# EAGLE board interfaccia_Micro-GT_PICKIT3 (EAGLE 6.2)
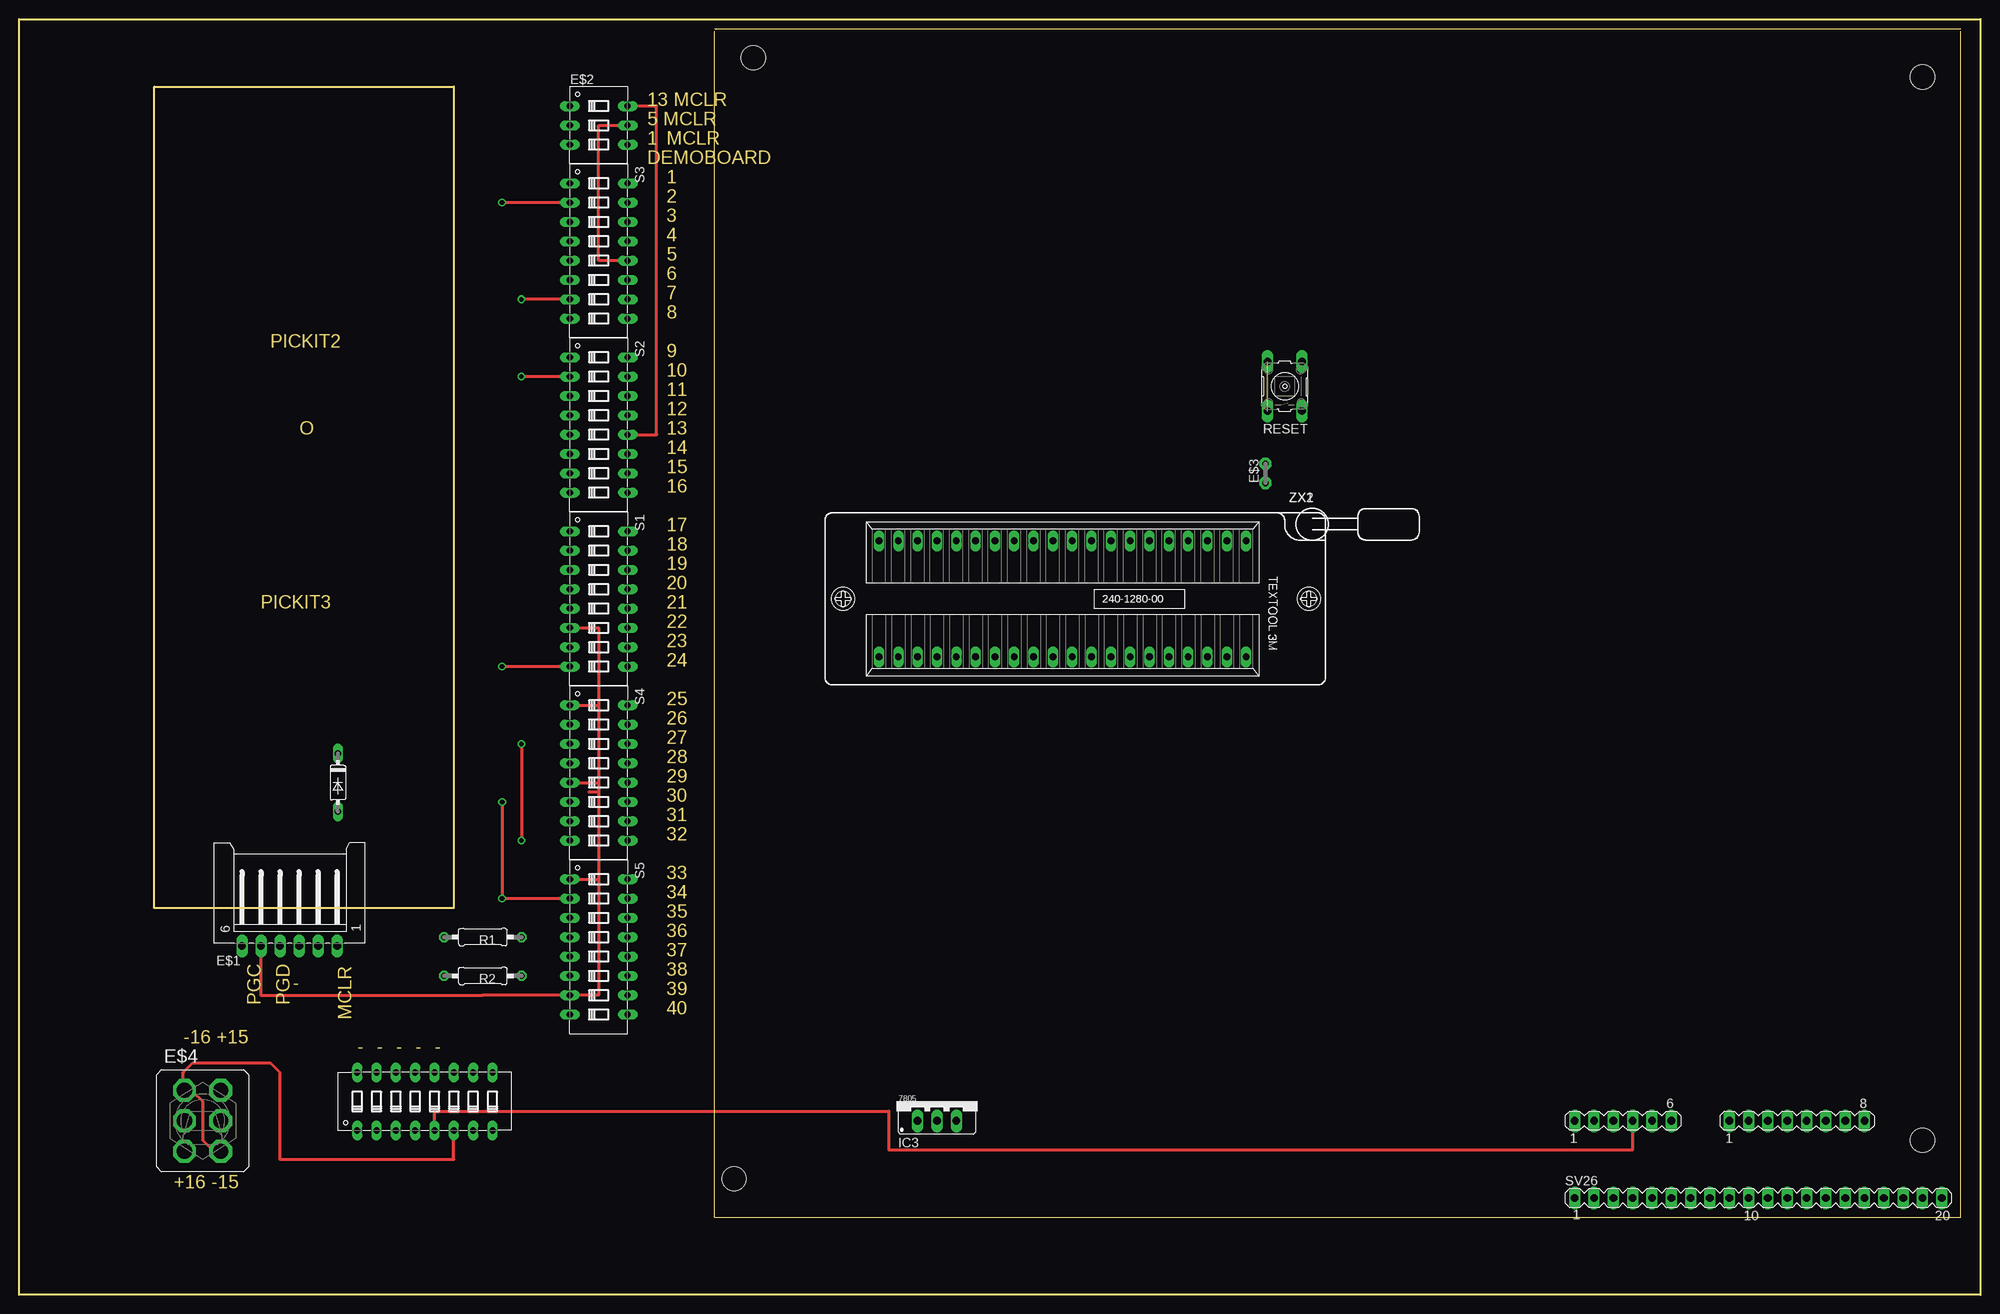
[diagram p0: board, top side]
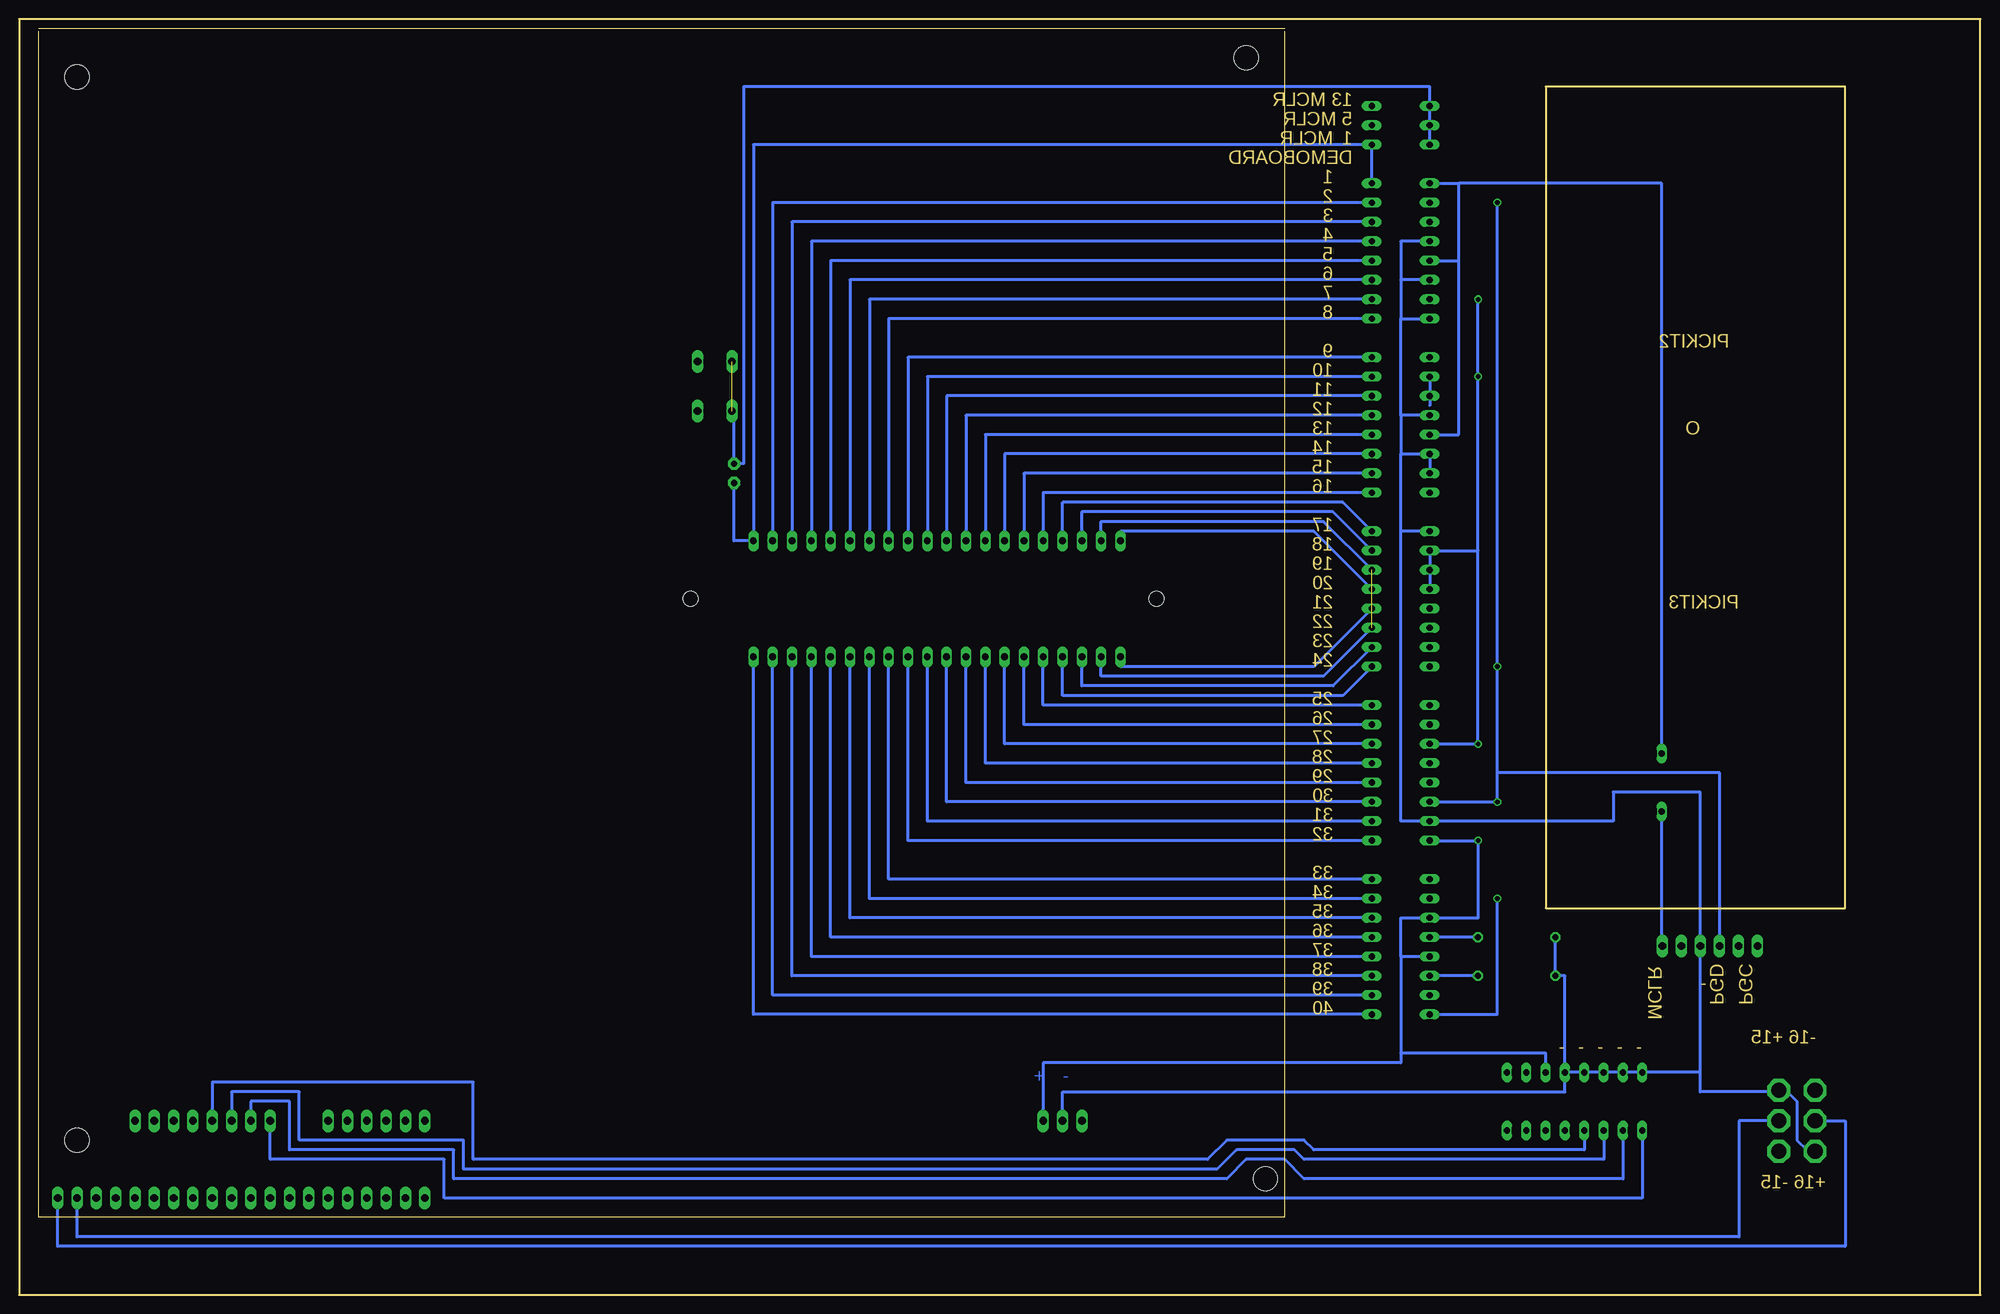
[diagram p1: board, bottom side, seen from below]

Size 257.81 x 167.64 mm. Coordinates in mm from the lower left corner, seen from the top.
Outline: 91.44,10.16 255.25,10.16 255.25,166.04
Outline: 91.42,10.16 91.42,166.04
Outline: 91.44,166.37 255.25,166.37
Outline: 0,0 0,167.64 257.81,167.64 257.81,0 0,0
Outline: 17.78,50.8 17.78,158.75 57.15,158.75 57.15,50.8 17.78,50.8
Copper layers (1*16): Top 0.035mm / dielectric 1.5mm / Bottom 0.035mm
Design rules: minimum track width 10mil, minimum drill 24mil, track to track 8mil, track to pad 8mil, pad to pad 8mil, via to via 8mil, smd to smd 8mil, copper to edge 40mil, drill to drill 8mil, minimum pad ring 10mil, minimum via ring 8mil, stop-mask expansion 4mil, vias tented up to drill 0mil, thermal gap 10mil
Holes 3.2 mm at 250.19,160.02 250.19,20.32 93.98,15.24 96.52,162.56

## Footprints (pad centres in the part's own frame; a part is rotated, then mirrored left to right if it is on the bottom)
DO35-7 = drill 0.813 long: A 3.81,0; C -3.81,0
L06P = drill 1.016 long: 1 6.25,-6.25; 2 3.75,-6.25; 3 1.25,-6.25; 4 -1.25,-6.25; 5 -3.75,-6.25; 6 -6.25,-6.25
DIP03YL = drill 0.813 long: 1 -2.54,-3.81; 2 0,-3.81; 3 2.54,-3.81; 4 2.54,3.81; 5 0,3.81; 6 -2.54,3.81
03 = drill 0.813 pad 1.6 octagon: 1 0,0; 2 2.54,0
320-938 = drill 2.007 octagon: 1 -2.388,4.013; 2 -2.388,0; 3 -2.388,-4.013; 4 2.388,4.013; 5 2.388,0; 6 2.388,-4.013
78XXS = drill 1.016 long: GND 0,-2.54; IN -2.54,-2.54; OUT 2.54,-2.54
0207/10 = drill 0.813 octagon: 1 -5.08,0; 2 5.08,0
B3F-10XX = drill 1.016 long: 1 -3.251,2.261; 2 3.251,2.261; 3 -3.251,-2.261; 4 3.251,-2.261
DIP08YL = drill 0.813 long: 1 -8.89,-3.81; 2 -6.35,-3.81; 3 -3.81,-3.81; 4 -1.27,-3.81; 5 1.27,-3.81; 6 3.81,-3.81; 7 6.35,-3.81; 8 8.89,-3.81; 9 8.89,3.81; 10 6.35,3.81; 11 3.81,3.81; 12 1.27,3.81; 13 -1.27,3.81; 14 -3.81,3.81; 15 -6.35,3.81; 16 -8.89,3.81
MA20-1 = drill 1.016 long: 1 -24.13,0; 2 -21.59,0; 3 -19.05,0; 4 -16.51,0; 5 -13.97,0; 6 -11.43,0; 7 -8.89,0; 8 -6.35,0; 9 -3.81,0; 10 -1.27,0; 11 1.27,0; 12 3.81,0; 13 6.35,0; 14 8.89,0; 15 11.43,0; 16 13.97,0; 17 16.51,0; 18 19.05,0; 19 21.59,0; 20 24.13,0
MA06-1 = drill 1.016 long: 1 -6.35,0; 2 -3.81,0; 3 -1.27,0; 4 1.27,0; 5 3.81,0; 6 6.35,0
MA08-1 = drill 1.016 long: 1 -8.89,0; 2 -6.35,0; 3 -3.81,0; 4 -1.27,0; 5 1.27,0; 6 3.81,0; 7 6.35,0; 8 8.89,0
240-1280-00-0602J = drill 0.9 long: 1 -24.13,-7.62; 2 -21.59,-7.62; 3 -19.05,-7.62; 4 -16.51,-7.62; 5 -13.97,-7.62; 6 -11.43,-7.62; 7 -8.89,-7.62; 8 -6.35,-7.62; 9 -3.81,-7.62; 10 -1.27,-7.62; 11 1.27,-7.62; 12 3.81,-7.62; 13 6.35,-7.62; 14 8.89,-7.62; 15 11.43,-7.62; 16 13.97,-7.62; 17 16.51,-7.62; 18 19.05,-7.62; 19 21.59,-7.62; 20 24.13,-7.62; 21 24.13,7.62; 22 21.59,7.62; 23 19.05,7.62; 24 16.51,7.62; 25 13.97,7.62; 26 11.43,7.62; 27 8.89,7.62; 28 6.35,7.62; 29 3.81,7.62; 30 1.27,7.62; 31 -1.27,7.62; 32 -3.81,7.62; 33 -6.35,7.62; 34 -8.89,7.62; 35 -11.43,7.62; 36 -13.97,7.62; 37 -16.51,7.62; 38 -19.05,7.62; 39 -21.59,7.62; 40 -24.13,7.62 | hole 2: 28.86,0; -32.36,0

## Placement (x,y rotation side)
D1  1N4007  [DO35-7]  41.91,67.31 270 top
E$1  [L06P]  35.56,52.07 0 top
E$2  [DIP03YL]  76.2,153.67 270 top
E$3  [03]  163.83,106.68 90 top
E$4  [320-938]  24.13,22.86 0 top
IC3  [78XXS]  120.65,25.4 0 top
R1  1K  [0207/10]  60.96,46.99 0 top
R2  1K  [0207/10]  60.96,41.91 0 top
RESET  [B3F-10XX]  166.37,119.38 90 top
S1  [DIP08YL]  76.2,91.44 270 top
S2  [DIP08YL]  76.2,114.3 270 top
S3  [DIP08YL]  76.2,137.16 270 top
S4  [DIP08YL]  76.2,68.58 270 top
S5  [DIP08YL]  76.2,45.72 270 top
S6  [DIP08YL]  53.34,25.4 0 top
SV26  [MA20-1]  228.6,12.7 0 top
SV27  [MA06-1]  210.82,22.86 0 top
SV28  [MA08-1]  233.68,22.86 0 top
ZX1  240-1280-00-0602J  [240-1280-00-0602J]  137.16,91.44 180 top
ZX2  240-1280-00-0602J  [240-1280-00-0602J]  137.16,91.44 180 top

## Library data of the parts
D1 = diode
E$1 = con-amp-mt
E$2 S1-S6 = switch-dil
E$3 = jumper
E$4 = switch
IC3 = v-reg
R1 R2 = resistor
RESET = switch-omron
SV26-SV28 = con-lstb
ZX1 ZX2 = con-3m

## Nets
N$87: RESET.1 RESET.2
N$124: ZX2.18
N$125: ZX2.23
N$128: ZX2.26
S$1: S5.9 ZX1.40
S$2: S5.10
S$3: S5.11 ZX1.38
S$4: S5.12 ZX1.37
S$5: S5.13 ZX1.36
S$6: S5.14 ZX1.35
S$7: S5.15 ZX1.34
S$8: S5.16 ZX1.33
S$9: S4.9 ZX1.32
S$10: S4.10 ZX1.31
S$12: S4.11 ZX1.30
S$13: S4.12 ZX1.29
S$14: S4.13 ZX1.28
S$15: S4.14 ZX1.27
S$16: S4.15 ZX1.26
S$18: S4.16 ZX1.25
S$19: ZX1.17
S$20: S1.10 ZX1.23
S$21: S1.11 ZX1.19 ZX1.22
S$22: S1.12 ZX1.20 ZX1.21
S$23: ZX1.18
S$24: S2.9 ZX1.16
S$25: S2.10 ZX1.15
S$26: S2.11 ZX1.14
S$27: E$2.6 S2.12 ZX1.13
S$28: S2.13 ZX1.12
S$29: S2.14 ZX1.11
S$30: S2.15 ZX1.10
S$31: S2.16 ZX1.9
S$32: S3.9 ZX1.8
S$33: S3.10 ZX1.7
S$34: S3.11 ZX1.6
S$35: E$2.5 S3.12 ZX1.5
S$36: S3.13 ZX1.4
S$37: S3.14 ZX1.3
S$38: S3.15 ZX1.2
S$39: S6.5 SV27.4
S$40: S3.5
S$41: D1.C S2.5 S3.1
S$43: R1.2 S5.4
S$44: R2.2 S5.6
S$46: E$2.1 E$2.3 E$3.2
S$47: S1.9 ZX1.24
S$48: IC3.OUT S1.2 S1.4 S2.2 S3.7 S4.3 S4.8 S5.3 S5.5 S6.11
S$49: S1.8 S3.2 S4.6 S5.2 S5.8
S$50: S1.6 S4.1
S$51: IC3.GND R1.1 R2.1 S1.1 S2.4 S2.6 S2.7 S3.4 S3.6 S3.8 S4.7 S6.12 S6.16
S$52: S4.5 S5.1 S5.7
S$53: E$2.4 E$3.1 S3.16 ZX1.1
S$56: S6.6
S$57: S6.1 SV28.1
S$58: S6.2 SV28.2
S$59: S6.3 SV28.3
S$60: S6.4 SV28.4
S$61: SV26.19
S$62: SV26.20

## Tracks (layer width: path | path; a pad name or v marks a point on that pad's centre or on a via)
N$87  (1 unrouted)
S$1
  Bottom 0.406: S5.9 161.29,36.83 ZX1.40
S$2
  Bottom 0.406: S5.10 158.75,39.37 158.75,83.82
S$3
  Bottom 0.406: S5.11 156.21,41.91 ZX1.38
S$4
  Bottom 0.406: S5.12 153.67,44.45 ZX1.37
S$5
  Bottom 0.406: S5.13 151.13,46.99 ZX1.36
S$6
  Bottom 0.406: S5.14 148.59,49.53 ZX1.35
S$7
  Bottom 0.406: S5.15 146.05,52.07 ZX1.34
S$8
  Bottom 0.406: S5.16 143.51,54.61 ZX1.33
S$9
  Bottom 0.406: S4.9 140.97,59.69 ZX1.32
S$10
  Bottom 0.406: S4.10 138.43,62.23 ZX1.31
S$12
  Bottom 0.406: S4.11 135.89,64.77 ZX1.30
S$13
  Bottom 0.406: S4.12 133.35,67.31 ZX1.29
S$14
  Bottom 0.406: S4.13 130.81,69.85 ZX1.28
S$15
  Bottom 0.406: S4.14 128.27,72.39 ZX1.27
S$16
  Bottom 0.406: S4.15 125.73,74.93 ZX1.26
S$18
  Bottom 0.406: S4.16 123.19,77.47 ZX1.25
S$19
  Bottom 0.406: 80.01,100.33 83.82,104.14 120.65,104.14 ZX1.17
S$20
  Bottom 0.406: S1.10 85.09,80.01 118.11,80.01 ZX1.23
S$21  (1 unrouted)
  Bottom 0.406: S1.11 86.36,81.28 115.57,81.28 ZX1.22 | 80.01,95.25 86.36,101.6 115.57,101.6 ZX1.19
S$22  (1 unrouted)
  Bottom 0.406: S1.12 87.63,82.55 113.03,82.55 ZX1.21 | 80.01,92.71 87.63,100.33 113.03,100.33 ZX1.20
S$23
  Bottom 0.406: 80.01,97.79 85.09,102.87 118.11,102.87 ZX1.18
S$24
  Bottom 0.406: S2.9 123.19,105.41 ZX1.16
S$25
  Bottom 0.406: S2.10 125.73,107.95 ZX1.15
S$26
  Bottom 0.406: S2.11 128.27,110.49 ZX1.14
S$27
  Top 0.406: S2.12 83.82,113.03 83.82,156.21 E$2.6
  Bottom 0.406: S2.12 130.81,113.03 ZX1.13
S$28
  Bottom 0.406: S2.13 133.35,115.57 ZX1.12
S$29
  Bottom 0.406: S2.14 135.89,118.11 ZX1.11
S$30
  Bottom 0.406: S2.15 138.43,120.65 ZX1.10
S$31
  Bottom 0.406: S2.16 140.97,123.19 ZX1.9
S$32
  Bottom 0.406: S3.9 143.51,128.27 ZX1.8
S$33
  Bottom 0.406: S3.10 146.05,130.81 ZX1.7
S$34
  Bottom 0.406: S3.11 148.59,133.35 ZX1.6
S$35
  Top 0.406: S3.12 76.2,135.89 76.2,153.67 E$2.5
  Bottom 0.406: S3.12 151.13,135.89 ZX1.5
S$36
  Bottom 0.406: S3.13 153.67,138.43 ZX1.4
S$37
  Bottom 0.406: S3.14 156.21,140.97 ZX1.3
S$38
  Bottom 0.406: S3.15 158.75,143.51 ZX1.2
S$39
  Top 0.406: S6.5 54.61,24.13 114.3,24.13 114.3,19.05 212.09,19.05 SV27.4
S$40
  Bottom 0.406: S3.5 68.58,135.89
S$41
  Bottom 0.406: S2.5 68.58,113.03 68.58,146.05 | S3.1 68.58,146.05 | D1.C 41.91,146.05 68.58,146.05
S$42
  Bottom 0.406: 41.91,45.72 41.91,62.23 41.91,63.5
S$43
  Bottom 0.406: R1.2 S5.4
S$44
  Bottom 0.406: R2.2 S5.6
S$46
  Bottom 0.406: 163.83,115.57 E$3.2 162.56,109.22 162.56,158.75 72.39,158.75 72.39,157.48 E$2.1 E$2.3
S$47
  Bottom 0.406: ZX1.24 120.65,78.74 83.82,78.74 S1.9
S$48  (via drill 0.6)
  Top 0.406: S3.7 v66.04,130.81 | S2.2 v66.04,120.65 | v66.04,72.39 v66.04,59.69
  Bottom 0.406: S6.11 57.15,31.75 76.2,31.75 | S5.5 76.2,44.45 | 76.2,44.45 76.2,49.53 S5.3 66.04,49.53 v66.04,59.69 S4.8 | S4.3 v66.04,72.39 66.04,97.79 | S1.4 S1.2 66.04,97.79 | 66.04,97.79 v66.04,120.65 v66.04,130.81 | S2.2 72.39,116.84 | 76.2,44.45 76.2,31.75 | 76.2,31.75 76.2,30.48 123.19,30.48 IC3.OUT
S$49  (via drill 0.6)
  Top 0.406: S3.2 v63.5,143.51 | S1.8 v63.5,82.55 | S5.2 v63.5,52.07 v63.5,64.77
  Bottom 0.406: S4.6 v63.5,64.77 63.5,68.58 | 63.5,68.58 v63.5,82.55 v63.5,143.51 | S5.8 63.5,36.83 v63.5,52.07 | 63.5,68.58 34.29,68.58 34.29,45.72
S$50
  Top 0.406: S1.6 76.2,87.63 76.2,77.47 | S4.1 76.2,77.47 | 76.2,77.47 76.2,76.2 76.2,66.04 74.93,66.04
S$51
  Bottom 0.406: IC3.GND 120.65,26.67 54.61,26.67 S6.12 | 36.83,29.21 36.83,66.04 48.26,66.04 48.26,62.23 S4.7 76.2,62.23 76.2,100.33 | S1.1 76.2,100.33 | S2.4 76.2,115.57 | S3.4 76.2,138.43 76.2,133.35 | 76.2,133.35 76.2,128.27 | 76.2,128.27 S3.8 | S3.6 76.2,133.35 | 76.2,115.57 76.2,128.27 | 76.2,115.57 76.2,110.49 | 76.2,110.49 S2.6 S2.7 | 76.2,100.33 76.2,110.49 | S6.12 S6.16 36.83,29.21 | S6.12 54.61,41.91 R2.1 R1.1 | 36.83,29.21 36.83,26.67 25.4,26.67 24.13,25.4 24.13,20.32 22.86,19.05 21.59,19.05
S$52
  Top 0.406: 31.75,45.72 31.75,39.37 60.96,39.37 62.23,39.37 S5.7 76.2,39.37 76.2,54.61 | S4.5 76.2,67.31 76.2,54.61 | S5.1 76.2,54.61
S$53
  Bottom 0.406: S3.16 E$2.4 161.29,151.13 ZX1.1 163.83,99.06 E$3.1
S$56
  Top 0.406: S6.6 57.15,17.78 34.29,17.78 34.29,29.21 33.02,30.48 22.86,30.48 21.59,29.21 21.59,26.67 22.86,26.67 24.13,25.4 24.13,20.32 25.4,19.05 26.67,19.05
S$57
  Bottom 0.406: S6.1 44.45,12.7 201.93,12.7 201.93,17.78 224.79,17.78 SV28.1
S$58
  Bottom 0.406: S6.2 46.99,15.24 88.9,15.24 91.44,17.78 96.52,17.78 99.06,15.24 200.66,15.24 200.66,19.05 222.25,19.05 222.25,25.4 227.33,25.4 SV28.2
S$59
  Bottom 0.406: S6.3 49.53,17.78 88.9,17.78 90.17,19.05 97.79,19.05 100.33,16.51 199.39,16.51 199.39,20.32 220.98,20.32 220.98,26.67 229.87,26.67 SV28.3
S$60
  Bottom 0.406: S6.4 52.07,19.05 87.63,19.05 88.9,20.32 99.06,20.32 101.6,17.78 198.12,17.78 198.12,27.94 232.41,27.94 SV28.4
S$61
  Bottom 0.406: 26.67,22.86 31.75,22.86 31.75,7.62 250.19,7.62 SV26.19
S$62
  Bottom 0.406: 21.59,22.86 17.78,22.86 17.78,6.35 252.73,6.35 SV26.20

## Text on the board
Bottom: - | +
Dimension: PICKIT2 | O | PICKIT3
tNames: 7805
Milling: 13 MCLR | 5 MCLR | 1 | MCLR | DEMOBOARD | 1 | 2 | 3 | 4 | 5 | 6 | 7 | 8 | 9 | 10 | 11 | 12 | 13 | 14 | 15 | 16 | 17 | 18 | 19 | 20 | 21 | 22 | 23 | 24 | 25 | 26 | 27 | 28 | 29 | 30 | 31 | 32 | 33 | 34 | 35 | 36 | 37 | MCLR | - | 38 | 39 | PGC | PGD | 40 | -16 +15 | - | - | - | - | - | +16 -15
